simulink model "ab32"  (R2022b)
settings: Solver=FixedStepAuto  StartTime=0.0  StopTime=1  FixedStep=0.001  RelTol=1e-3
libraries: simulink x1

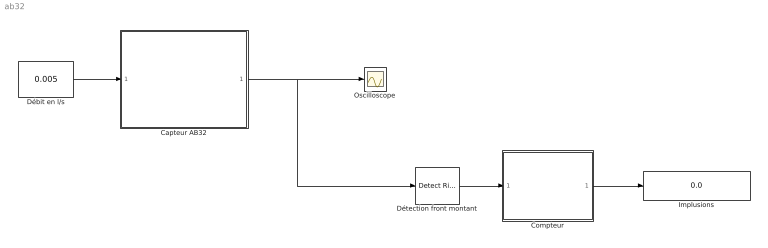
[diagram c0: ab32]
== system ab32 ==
  Capteur AB32 : Subsystem
  Compteur : MATLAB Function  TreatAsAtomicUnit=on
  Débit en l/s : Constant  Value=0.005
  Détection front montant : simulink/Logic and Bit Operations/Detect Rise Positive  vinit=0  OutDataTypeStr=boolean
  Implusions : Display
  Oscilloscope : Scope
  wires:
  Compteur/1(count) -> Implusions/1
  Détection front montant/1 -> Compteur/1(pulse)
  Capteur AB32/1(y) -> Oscilloscope/1, Détection front montant/1
  Débit en l/s/1 -> Capteur AB32/1(In1)

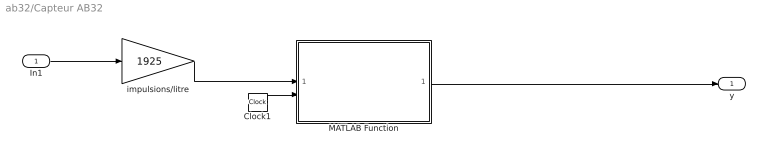
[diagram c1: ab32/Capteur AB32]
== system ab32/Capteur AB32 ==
  In1 : Inport
  Clock1 : Clock
  MATLAB Function : MATLAB Function  TreatAsAtomicUnit=on
  impulsions/litre : Gain  Gain=1925
  y : Outport
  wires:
  Clock1/1 -> MATLAB Function/2(t)
  impulsions/litre/1 -> MATLAB Function/1(f)
  In1/1 -> impulsions/litre/1
  MATLAB Function/1(y) -> y/1

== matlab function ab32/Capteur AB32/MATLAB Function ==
function y = pulse_signal(f, t)
% Entrée : f (fréquence en Hz), t (temps de simulation)
% Sortie : y (signal carré 0/1)
T = 1/f; % Période
y = mod(t, T) < T/2; % Génère un signal carré (1 si t mod T < T/2, 0 sinon)
end

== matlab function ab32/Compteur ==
function count = impulse_counter(pulse)
%#codegen
persistent c
if isempty(c)
    c = 0;
end
if pulse
    c = c + 1;
end
count = c;
